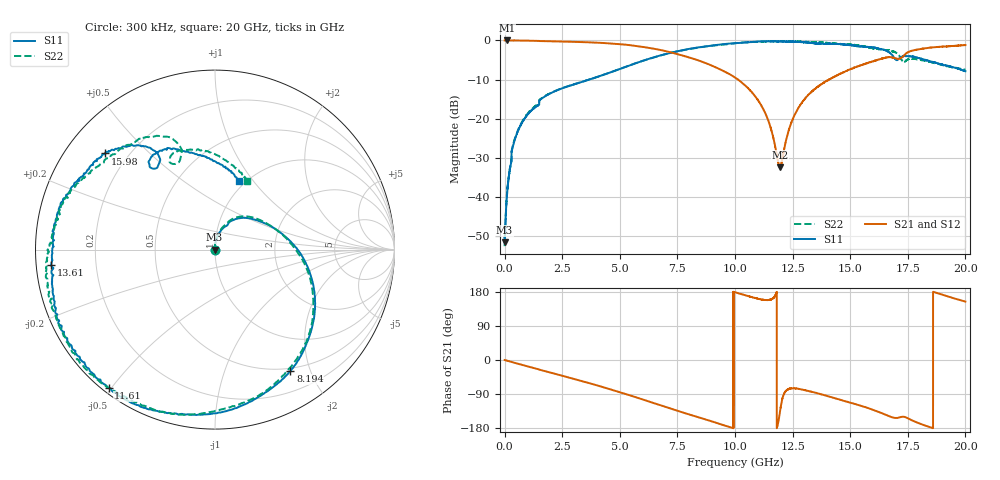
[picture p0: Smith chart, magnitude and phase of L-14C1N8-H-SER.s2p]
!{L-14C1N8}
!Johanson Technology Inc.
!www.johansontechnology.com
!Test Board Conditions:
!Substrate Type  RO4350B
!Substrate Thickness  20 mil
!Substrate Dk  3.66
!TL Type: GCPW
!TL Trace Width  36 mil
!TL Gap  12 mil
!Electrode orientation  Horizontal
!DUT TOPOLOGY	SERIES
!Mounting Pad LxW  26x36 mil
! Created Sun Jun 20 12:54:18 2021
# hz S ma R 50
! 2 Port Network Data from SP1.SP block
! freq  magS11  angS11  magS21  angS21  magS12  angS12  magS22  angS22
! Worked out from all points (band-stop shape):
!   20001 points, 300 kHz to 20 GHz, reference 50 ohm
!   highest |S21| = -0.01 dB at 108.3 MHz (marker M1); lowest = -32.4 dB at 11.96 GHz (marker M2)
!   |S21| within 3 dB of the highest: start of sweep to 7.186 GHz; 17.51 GHz to end of sweep
!   lowest |S11| = -51.6 dB at 300 kHz (marker M3), VSWR 1.01, Z = 49.7 + j0.0191 ohm
!   |S11| at or under -10 dB: start of sweep to 3.67 GHz; 3.670402 GHz to 3.67314 GHz (2.737 MHz wide, 0.0746 % of centre); 3.673437 GHz to 3.677015 GHz (3.578 MHz wide, 0.0974 % of centre)
!   |S22| runs from -52.6 to -0.1 dB; largest |S21 - S12| = 0.019
!   S11 on the Smith chart (normalised r, x): 300 kHz: 0.99, +0.00; 8.194 GHz: 0.46, -1.71; 11.61 GHz: 0.02, -0.49; 13.61 GHz: 0.04, -0.05; 15.98 GHz: 0.12, +0.37; 20 GHz: 0.94, +0.85
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300000  0.002644 175.8  0.9983 -0.0  0.9963 -0.0  0.002349 -178.1
1.083e8  0.01131 100.9  0.9983 -1.8  0.9966 -1.8  0.01152 98.7
4.003e8  0.04899 84.1  0.9976 -6.9  0.9973 -6.9  0.05052 84.5
8.283e8  0.09644 75.6  0.9946 -14.0  0.9938 -14.0  0.09833 76.7
1.6573e9  0.1846 60.3  0.9794 -27.9  0.9797 -27.9  0.1865 62.2
3.3343e9  0.2935 32.7  0.9521 -55.4  0.9519 -55.4  0.2942 35.1
5.0303e9  0.4352 4.1  0.894 -85.7  0.8922 -85.6  0.434 2.6
6.6673e9  0.6314 -27.9  0.7643 -117.6  0.7613 -117.5  0.6296 -29.6
8.1943e9  0.7963 -58.1  0.5824 -147.2  0.5791 -146.6  0.7891 -59.9
1.00003e10  0.9208 -93.8  0.3356 178.8  0.3361 179.1  0.92 -95.7
1.09923e10  0.9663 -114.6  0.1731 161.8  0.1756 162.1  0.9576 -116.4
1.16093e10  0.9717 -127.6  0.06612 161.5  0.06635 161.7  0.9765 -131.5
1.19553e10  0.9681 -136.6  0.02405 -135.3  0.02447 -135.7  0.9816 -139.4
1.25393e10  0.9621 -150.9  0.1039 -74.8  0.1056 -75.9  0.9668 -152.8
1.33343e10  0.9286 -168.5  0.2221 -84.0  0.222 -84.8  0.9542 -169.0
1.36123e10  0.9166 -174.7  0.2579 -88.5  0.2578 -89.3  0.9441 -173.7
1.59773e10  0.8133 138.8  0.5407 -131.3  0.5388 -131.4  0.795 142.9
1.66673e10  0.7089 125.7  0.6119 -147.5  0.609 -145.9  0.7497 125.1
1.71883e10  0.6089 127.2  0.5905 -150.6  0.5873 -149.9  0.5935 108.6
1.75143e10  0.6303 119.5  0.7079 -154.2  0.7079 -154.0  0.5726 115.9
1.85763e10  0.5309 98.5  0.813 -179.6  0.8167 -179.4  0.5235 87.9
2e10  0.4036 70.5  0.8722 154.1  0.8722 154.6  0.422 64.6
